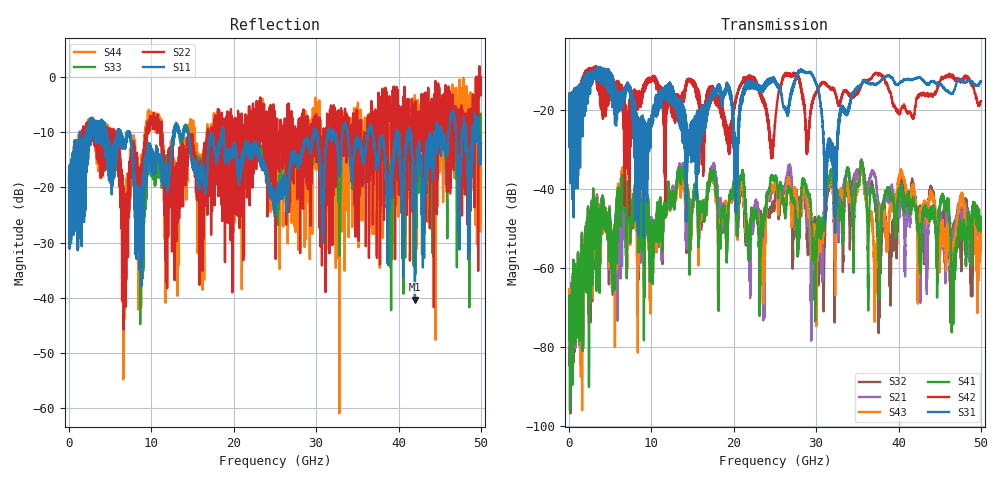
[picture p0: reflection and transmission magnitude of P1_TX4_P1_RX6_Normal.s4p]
!Keysight Technologies,N5225B,MY57041031,A.13.20.10
!Date: Friday, May 31, 2019 11:22:31
!Correction: S11(Full 4 Port(1,2,3,4))
!S12(Full 4 Port(1,2,3,4))
!S13(Full 4 Port(1,2,3,4))
!S14(Full 4 Port(1,2,3,4))
!S21(Full 4 Port(1,2,3,4))
!S22(Full 4 Port(1,2,3,4))
!S23(Full 4 Port(1,2,3,4))
!S24(Full 4 Port(1,2,3,4))
!S31(Full 4 Port(1,2,3,4))
!S32(Full 4 Port(1,2,3,4))
!S33(Full 4 Port(1,2,3,4))
!S34(Full 4 Port(1,2,3,4))
!S41(Full 4 Port(1,2,3,4))
!S42(Full 4 Port(1,2,3,4))
!S43(Full 4 Port(1,2,3,4))
!S44(Full 4 Port(1,2,3,4))
!S4P File: Measurements: <S11,S12,S13,S14>,
!<S21,S22,S23,S24>,
!<S31,S32,S33,S34>,
!<S41,S42,S43,S44>:
# Hz S  dB  R 50.0
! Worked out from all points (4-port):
!   5000 points, 10 MHz to 50 GHz, reference 50 ohm
!   strongest paths, dB at 10 MHz, 12.51 GHz, 25.01 GHz, 37.51 GHz, 50 GHz:
!     S31: -19.6, -17.6, -12.9, -13.1, -12.6
!     S42: -19.4, -15.6, -23.0, -10.9, -17.7
!     S41: -68.8, -41.5, -36.7, -50.9, -49.1
!     S43: -72.1, -41.0, -38.6, -54.1, -51.6
!     S21: -80.7, -40.7, -38.8, -42.6, -53.5
!     S32: -67.4, -40.4, -42.4, -69.3, -51.6
!   lowest |S11| = -40.4 dB at 41.99 GHz (marker M1), VSWR 1.02, Z = 51 - j0.191 ohm
!   |S11| at or under -10 dB: 7.336 GHz to 12.7 GHz (5.362 GHz wide, 53.5 % of centre); 14.42 GHz to 18.57 GHz (4.156 GHz wide, 25.2 % of centre); 18.74 GHz to 29.76 GHz (11.02 GHz wide, 45.4 % of centre)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
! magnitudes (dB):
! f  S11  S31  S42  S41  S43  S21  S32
! 10 MHz  -19.5  -19.6  -19.4  -68.8  -72.1  -80.7  -67.4
! 6.59 GHz  -12.1  -15.0  -19.7  -37.7  -35.5  -44.5  -40.0
! 20.25 GHz  -13.1  -33.9  -17.4  -41.7  -43.6  -41.7  -42.7
! 29.18 GHz  -13.0  -10.2  -23.0  -41.8  -46.1  -49.2  -52.1
! 32.24 GHz  -10.4  -35.4  -15.2  -43.1  -51.2  -42.4  -73.7
! 41.99 GHz  -40.4  -11.9  -19.5  -44.0  -43.2  -41.9  -42.1
! 50 GHz  -12.0  -12.6  -17.7  -49.1  -51.6  -53.5  -51.6
